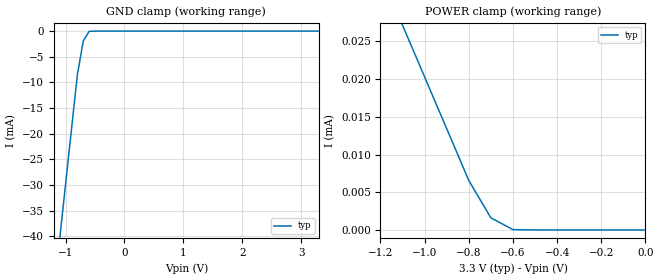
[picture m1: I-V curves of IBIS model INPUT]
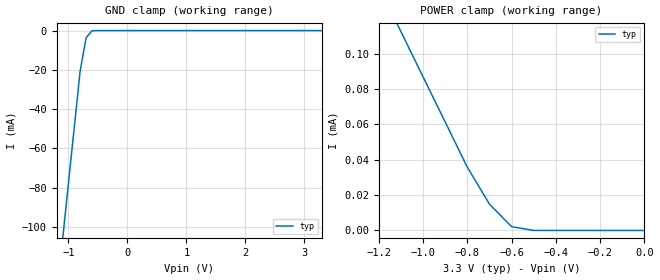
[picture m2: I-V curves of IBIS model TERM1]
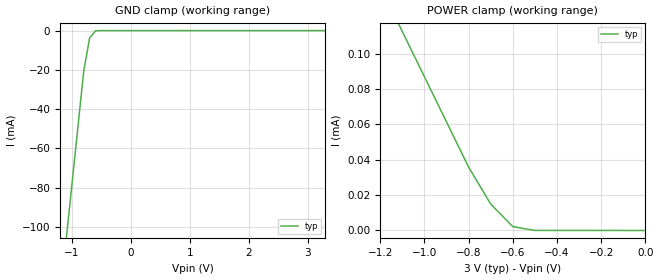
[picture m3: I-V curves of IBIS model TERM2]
| IBIS file max4906f.ibs created at Maxim Integrated Products
[IBIS ver]   3.2
[File name]   max4906f.ibs
[File Rev]   1.0
[Date]   May 26, 2006
[Source]   Data was acquired from HSpice simulations.
[Notes]   This is a dual SPDT analog switch. This IBIS model is not
   verified using any software.
[Disclaimer] Maxim Integrated Products hereby grants the user of this
   IBIS model a non-exclusive, nontransferable license to use
   this IBIS model under the following terms. Before using
   this IBIS model, the user should read this license. If the
   user does not accept these terms, the IBIS model should be
   returned to Maxim Integrated Products within 30 days.
   The user is granted this license only to use the IBIS model
   and is not granted rights to sell, load, rent, lease or
   license the IBIS model in whole or in part, or in modified
   form to anyone other than user. User may modify the IBIS
   model to suit its specific applications but rights to
   derivative works and such modifications shall belong to
   Maxim Integrated Products. This IBIS model is provided on
   an "AS IS" basis and Maxim Integrated Products makes
   absolutely no warranty with respect to the information
   contained herein.MAXIM INTEGRATED PRODUCTS DISCLAIMS AND
   CUSTOMER WAIVES ALL WARRANTIES, EXPRESS OR IMPLIED,
   INCLUDING WARRANTIES OF MERCHANTABILITY OR FITNESS FOR A
   PARTICULAR PURPOSE. The entire risk as to quality and
   performance is with the Customer. ACCORDINGLY, IN NO EVENT
   SHALL THE COMPANY BE LIABLE FOR ANY DAMAGES, WHETHER IN
   CONTRACT OR TORT,INCLUDING ANY LOST PROFITS OR OTHER
   INCIDENTAL, CONSEQUENTIAL, EXEMPLARY, OR PUNITIVE DAMAGES
   ARISING OUT OF THE USE OR APPLICATION OF THE IBIS model
   provided in this package.Further, Maxim Integrated Products
   reserves the right to make changes without notice to any
   product herein to improve reliability, function, or design.
   Maxim Integrated Products does not convey any license under
   patent rights or any other intellectual property rights,
   including those of third parties.
   Maxim Integrated Products is not obligated to provide
   maintenance or support for the licensed IBIS model.
[Copyright]   Copyright of Maxim Integrated Products.
|   Component MAX4906F
[Component]   MAX4906F
[Manufacturer]   Maxim Integrated Products
[Package]
|variable   typ   min   max
R_pkg   34.430E-03   NA   NA
L_pkg   0.502E-09   NA   NA
C_pkg   0.188E-12   NA   NA
[Pin]  signal_name   model_name   R_pin   L_pin   C_pin
1   IN   INPUT
2   SHDN   INPUT
3   GND   GND
4   COM1   TERM2
5   COM2   TERM2
6   NO2   TERM1
7   NO1   TERM1
8   NC2   TERM1
9   NC1   TERM1
10   V+   POWER
[Series Switch Groups]
On 1 /
Off 2 /
[Series Pin Mapping]   pin_2   model_name  function_table_group
4   9   SWITCH1   1
4   7   SWITCH1   2
5   8   SWITCH1   1
5   6   SWITCH1   2
|   Switch Characteristics
[Model] SWITCH1
Model_type Series_switch
C_comp   9pF   NA   NA
[Temperature Range]   25   85   -40
[Voltage Range]   3.30V   3.00V   3.60V
[POWER Clamp Reference]   3.30V   3.00V   3.60V
[GND Clamp Reference]   0.00V   0.00V   0.00V
[On]
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[Off]
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| Models and submodels in the file (4): INPUT (Input), SWITCH1 (Series_switch), TERM1 (Terminator), TERM2 (Terminator)
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|   Switch Control Inputs
[Model] INPUT
|Signals   IN, SHDN
Model_type Input
Vinl = 0.40V
Vinh = 1.10V
C_comp   0.601pF   NA   NA
[Temperature Range]   25   85   -40
[Voltage Range]   3.30V   3.00V   3.60V
[POWER Clamp Reference]   3.30V   3.00V   3.60V
[GND Clamp Reference]   0.00V   0.00V   0.00V
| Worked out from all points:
|   GND clamp passes 1 mA (typ) near -0.65 V on its own axis
[POWER_clamp]
| Note that the [POWER_clamp] voltage table is referenced to Vcc
| and is calculated using Vtable=Vcc - Vmeasured.
|V(V)   I(typ)   I(min)  I(max)
-3.3V     198.1uA    NA         NA
-1.1V     27.13uA    NA         NA
-1V       20.28uA    NA         NA
-800mV    6.56uA     NA         NA
-700mV    1.607uA    NA         NA
-600mV    46.28nA    NA         NA
0V        -323.4pA   NA         NA
[GND_clamp]
| Note that the [GND_clamp] voltage table is referenced to Gnd.
|V(V)   I(typ)   I(min)  I(max)
-3.3V     -307.4mA   NA         NA
-1.1V     -40.46mA   NA         NA
-1V       -29.81mA   NA         NA
-800mV    -8.494mA   NA         NA
-700mV    -1.926mA   NA         NA
-600mV    -52.26uA   NA         NA
3.3V      347.5pA    NA         NA
|   Switch Inputs
[Model] TERM1
|Signals   NC1, NC2, NO1, NO2
Model_type Terminator
C_comp   4pF   NA   NA
[Temperature Range]   25   85   -40
[Voltage Range]   3.30V   3.00V   3.60V
[POWER Clamp Reference]   3.30V   3.00V   3.60V
[GND Clamp Reference]   0.00V   0.00V   0.00V
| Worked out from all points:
|   GND clamp passes 1 mA (typ) near -0.62 V on its own axis
[POWER_clamp]
| Note that the [POWER_clamp] voltage table is referenced to Vcc
| and is calculated using Vtable=Vcc - Vmeasured.
|V(V)   I(typ)   I(min)  I(max)
-3.3V     623.5uA    NA         NA
-1.2V     138uA      NA         NA
-1.1V     112.5uA    NA         NA
-800mV    35.82uA    NA         NA
-700mV    14.92uA    NA         NA
-600mV    2.181uA    NA         NA
-500mV    32.57nA    NA         NA
0V        -957.3pA   NA         NA
[GND_clamp]
| Note that the [GND_clamp] voltage table is referenced to Gnd.
|V(V)   I(typ)   I(min)  I(max)
-3.3V     -975.1mA   NA         NA
-1.1V     -107.1mA   NA         NA
-1V       -78.24mA   NA         NA
-800mV    -20.59mA   NA         NA
-700mV    -3.766mA   NA         NA
-600mV    -120.1uA   NA         NA
3.3V      912.3pA    NA         NA
|   Switch Common Inputs
[Model] TERM2
|Signals   COM1, COM2
Model_type Terminator
C_comp   5pF   NA   NA
[Temperature Range]   25   85   -40
[Voltage Range]   3.00V   2.70V   3.60V
[POWER Clamp Reference]   3.00V   2.70V   3.60V
[GND Clamp Reference]   0.00V   0.00V   0.00V
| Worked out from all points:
|   GND clamp passes 1 mA (typ) near -0.62 V on its own axis
[POWER_clamp]
| Note that the [POWER_clamp] voltage table is referenced to Vcc
| and is calculated using Vtable=Vcc - Vmeasured.
|V(V)   I(typ)   I(min)  I(max)
-3.3V     623.5uA    NA         NA
-1.2V     138uA      NA         NA
-1.1V     112.5uA    NA         NA
-800mV    35.82uA    NA         NA
-700mV    14.92uA    NA         NA
-600mV    2.181uA    NA         NA
-500mV    32.57nA    NA         NA
0V        -957.3pA   NA         NA
[GND_clamp]
| Note that the [GND_clamp] voltage table is referenced to Gnd.
|V(V)   I(typ)   I(min)  I(max)
-3.3V     -975.1mA   NA         NA
-1.1V     -107.1mA   NA         NA
-1V       -78.24mA   NA         NA
-800mV    -20.59mA   NA         NA
-700mV    -3.766mA   NA         NA
-600mV    -120.1uA   NA         NA
3.3V      912.3pA    NA         NA
